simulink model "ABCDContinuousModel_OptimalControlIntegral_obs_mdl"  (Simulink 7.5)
settings: Solver=ode45  StartTime=0.0  StopTime=10.0  FixedStep=Ts  RelTol=1e-3
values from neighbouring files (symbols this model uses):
  H = Ki(n+1)    [TSC140415ProvaMatlab.m]
  K = Ki(1:n)    [TSC140415ProvaMatlab.m]
  L = -acker(A',C',[0 0 0])'    [TSC140415ProvaMatlab.m]
  n = 3    [TSC140415ProvaMatlab.m]
  tp = 2    [TSC140415ProvaMatlab.m]
  Ts = 0.05    [TSC140415ProvaMatlab.m]
  yp = 4    [TSC140415ProvaMatlab.m]
undefined symbols (not defined in the file or in its folder): A, B, C, DiscIntNeverNeededParam
libraries: cstblocks x1, simulink x1

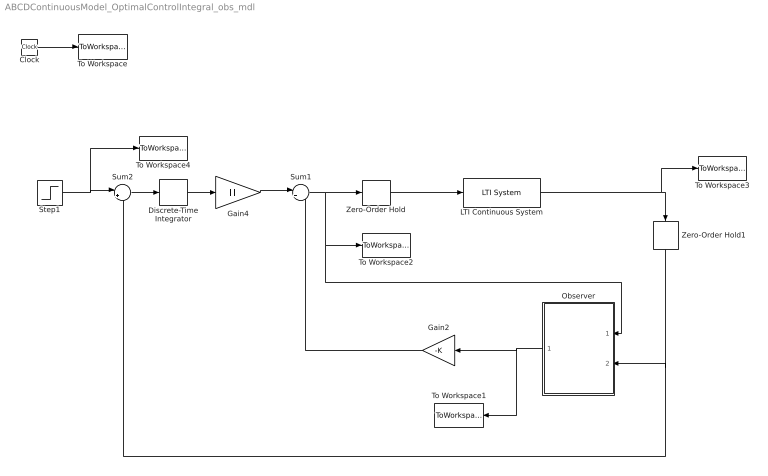
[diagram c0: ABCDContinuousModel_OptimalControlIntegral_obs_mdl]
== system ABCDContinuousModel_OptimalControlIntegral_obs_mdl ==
  Clock : Clock
  Discrete-Time Integrator : DiscreteIntegrator  SampleTime=Ts  OutDataType=sfix(16)  OutScaling=2^0  ICPrevOutput=DiscIntNeverNeededParam  ICPrevScaledInput=DiscIntNeverNeededParam
  Gain2 : Gain  Gain=-K  Multiplication=Matrix(K*u)  ParameterDataType=sfix(16)  ParameterScaling=2^0  OutDataType=sfix(16)  OutScaling=2^0
  Gain4 : Gain  Gain=H  Multiplication=Matrix(K*u)  ParameterDataType=sfix(16)  ParameterScaling=2^0  OutDataType=sfix(16)  OutScaling=2^0
  LTI Continuous System : cstblocks/LTI System  SystemSampleTime=-1  sys=sys  IC=X0
  Observer : Subsystem
  Step1 : Step  Time=tp  After=yp  SampleTime=0
  Sum1 : Sum  Inputs=|++  OutDataType=sfix(16)  OutScaling=2^0
  Sum2 : Sum  Inputs=|+-  OutDataType=sfix(16)  OutScaling=2^0
  To Workspace : ToWorkspace  VariableName=time  SampleTime=-1  SaveFormat=Array
  To Workspace1 : ToWorkspace  VariableName=Xs  SampleTime=-1  SaveFormat=Array
  To Workspace2 : ToWorkspace  VariableName=u  SampleTime=-1  SaveFormat=Array
  To Workspace3 : ToWorkspace  VariableName=y  SampleTime=-1  SaveFormat=Array
  To Workspace4 : ToWorkspace  VariableName=yd  SampleTime=-1  SaveFormat=Array
  Zero-Order Hold : ZeroOrderHold  SampleTime=Ts
  Zero-Order Hold1 : ZeroOrderHold  SampleTime=Ts
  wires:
  Gain4/1 -> Sum1/1
  Step1/1 -> To Workspace4/1, Sum2/1
  Gain2/1 -> Sum1/2
  Sum1/1 -> To Workspace2/1, Observer/1(u), Zero-Order Hold/1
  Clock/1 -> To Workspace/1
  Discrete-Time Integrator/1 -> Gain4/1
  Sum2/1 -> Discrete-Time Integrator/1
  Observer/1(Out1) -> Gain2/1, To Workspace1/1
  Zero-Order Hold/1 -> LTI Continuous System/1
  Zero-Order Hold1/1 -> Observer/2(y), Sum2/2
  LTI Continuous System/1 -> Zero-Order Hold1/1, To Workspace3/1

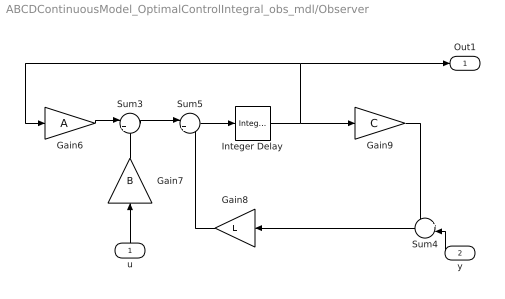
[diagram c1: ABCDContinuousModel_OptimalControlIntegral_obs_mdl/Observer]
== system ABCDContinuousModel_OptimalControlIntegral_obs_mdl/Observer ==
  u : Inport
  y : Inport  Port=2
  Gain6 : Gain  Gain=A  Multiplication=Matrix(K*u)  ParameterDataType=sfix(16)  ParameterScaling=2^0  OutDataType=sfix(16)  OutScaling=2^0
  Gain7 : Gain  Gain=B  Multiplication=Matrix(K*u)  ParameterDataType=sfix(16)  ParameterScaling=2^0  OutDataType=sfix(16)  OutScaling=2^0
  Gain8 : Gain  Gain=L  Multiplication=Matrix(K*u)  ParameterDataType=sfix(16)  ParameterScaling=2^0  OutDataType=sfix(16)  OutScaling=2^0
  Gain9 : Gain  Gain=C  Multiplication=Matrix(K*u)  ParameterDataType=sfix(16)  ParameterScaling=2^0  OutDataType=sfix(16)  OutScaling=2^0
  Integer Delay : simulink/Discrete/Integer Delay  vinit=zeros(1,n)  samptime=Ts  NumDelays=1
  Sum3 : Sum  Inputs=|++  OutDataType=sfix(16)  OutScaling=2^0
  Sum4 : Sum  Inputs=+-  OutDataType=sfix(16)  OutScaling=2^0
  Sum5 : Sum  Inputs=|++  OutDataType=sfix(16)  OutScaling=2^0
  Out1 : Outport
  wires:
  Gain6/1 -> Sum3/1
  Integer Delay/1 -> Gain9/1, Gain6/1, Out1/1
  Gain7/1 -> Sum3/2
  Sum4/1 -> Gain8/1
  Gain9/1 -> Sum4/1
  Gain8/1 -> Sum5/2
  Sum3/1 -> Sum5/1
  Sum5/1 -> Integer Delay/1
  u/1 -> Gain7/1
  y/1 -> Sum4/2
